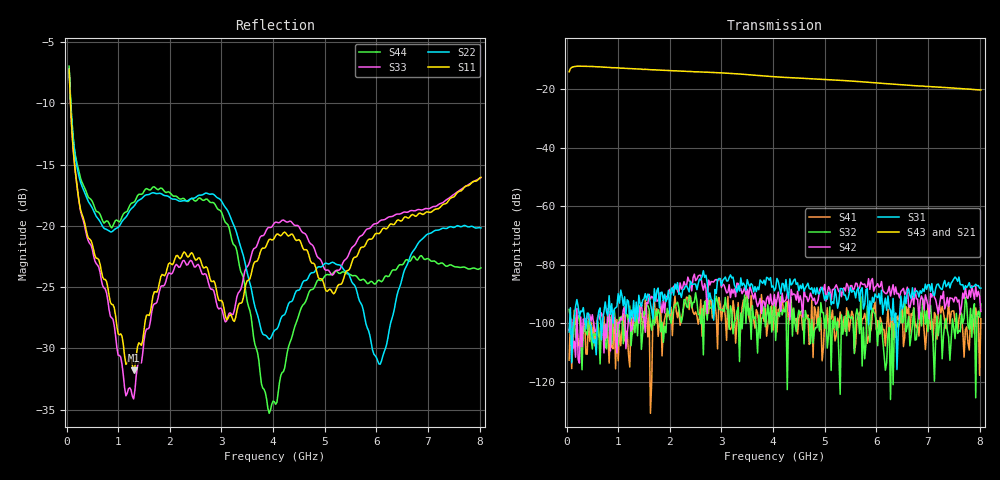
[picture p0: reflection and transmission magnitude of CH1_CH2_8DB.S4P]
!Agilent Technologies,E5071C,MY46316741,A.11.02
!Date: Thu May 28 14:26:45 2026
!Data & Calibration Information:
!1:CH1 INPUT 2:CH1 OUTPUT 3:CH2 INPUT 4:CH2 OUTPUT
!Freq	S11:SOLT4(ON)	S12:SOLT4(ON)	S13:SOLT4(ON)	S14:SOLT4(ON)
!	S21:SOLT4(ON)	S22:SOLT4(ON)	S23:SOLT4(ON)	S24:SOLT4(ON)
!	S31:SOLT4(ON)	S32:SOLT4(ON)	S33:SOLT4(ON)	S34:SOLT4(ON)
!	S41:SOLT4(ON)	S42:SOLT4(ON)	S43:SOLT4(ON)	S44:SOLT4(ON)
!PortZ  Port1:50+j0  Port2:50+j0  Port3:50+j0  Port4:50+j0
!Above PortZ is port z conversion or system Z0 setting when saving the data.
!When reading, reference impedance value at option line is always used.
# Hz S dB R 50
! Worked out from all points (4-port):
!   320 points, 50 MHz to 8.025 GHz, reference 50 ohm
!   strongest paths, dB at 50 MHz, 2.05 GHz, 4.05 GHz, 6.05 GHz, 8.025 GHz:
!     S43: -14.1, -13.7, -15.8, -18.0, -20.3
!     S21: -14.2, -13.9, -15.9, -18.0, -20.4
!     S31: -102.9, -87.7, -88.0, -89.8, -87.9
!     S42: -102.3, -89.2, -94.2, -87.6, -95.9
!     S32: -95.2, -96.9, -105.8, -99.1, -93.4
!     S41: -112.6, -104.2, -91.9, -103.8, -98.4
!   lowest |S11| = -31.8 dB at 1.3 GHz (marker M1), VSWR 1.05, Z = 47.9 - j1.34 ohm
!   |S11| at or under -10 dB: 76.94 MHz to end of sweep
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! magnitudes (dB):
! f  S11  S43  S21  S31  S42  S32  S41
! 50 MHz  -7.2  -14.1  -14.2  -102.9  -102.3  -95.2  -112.6
! 1.3 GHz  -31.8  -13.1  -13.2  -92.2  -96.4  -100.3  -100.7
! 3 GHz  -26.1  -14.5  -14.6  -87.1  -87.7  -95.3  -99.1
! 3.925 GHz  -21.1  -15.7  -15.7  -85.2  -93.3  -100.2  -96.8
! 4.875 GHz  -24.2  -16.6  -16.7  -89.8  -91.8  -98.2  -94.4
! 6.075 GHz  -20.6  -18.0  -18.0  -93.4  -87.4  -103.5  -97.9
! 8.025 GHz  -16.0  -20.3  -20.4  -87.9  -95.9  -93.4  -98.4
